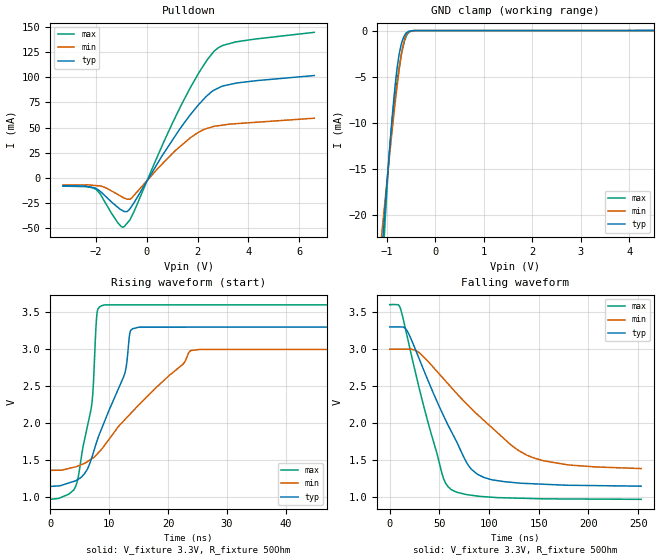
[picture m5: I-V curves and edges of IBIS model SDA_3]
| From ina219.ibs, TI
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|   3.3V SDA I/O_Open_drain Model
[Model] SDA_3   |Rload = 1k
Model_type I/O_open_drain
| Signals  SDA
Polarity   Non-Inverting
Enable   Active-Low
Vinl = 0.99
Vinh = 2.31
Vmeas = 1.65
Vref = 1.65
Cref = 0pF
Rref = 50
|   typ   min   max
|Average
C_comp   2.0039139E-10   2.3760390E-10   2.1698516E-10
|ON state
|C_comp   2.2433820e-12   2.5433970e-12   1.9431160e-12
|OFF state
|C_comp   3.9853940e-10   4.7266440e-10   4.7266440e-10
[Voltage Range]   3.3   3   3.6
[Temperature Range]   27   85   -25
[Pullup Reference]   3.3   3   3.6
[Pulldown Reference]   0   0   -0
[Power Clamp Reference]   3.3   3   3.6
[GND Clamp Reference]   0   0   0
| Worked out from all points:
|   slope of the pulldown table from 0 to 0.495 V, typ, clamps not added: 23.7 ohm
|   GND clamp passes 1 mA (typ) near -0.67 V on its own axis
|   falling waveform, V_fixture 3.3V, R_fixture 50Ohm: 20-80 % time 43.6ns typ, 72.7ns min, 30.1ns max; typ from 3.3 V to 1.15 V
|   rising waveform, V_fixture 3.3V, R_fixture 50Ohm: 20-80 % time 5.85ns typ, 11.5ns min, 2.43ns max; typ from 1.15 V to 3.3 V
[Pulldown]
|   Voltage   I(typ)   I(min)   I(max)
-3.3V     -7.794mA   -7.117mA   -8.174mA
-1.996V   -10.52mA   -7.627mA   -11.41mA
-1.14V    -29.25mA   -16.51mA   -44.63mA
-895.3mV  -33.38mA   -19.99mA   -48.61mA
-772.4mV  -33.44mA   -21.14mA   -45.1mA
-599.6mV  -28.41mA   -20.19mA   -38.58mA
630.8mV   22.96mA    14.44mA    33.51mA
1.346V    50.2mA     31.9mA     71.87mA
2.067V    73.55mA    45.72mA    105.3mA
2.644V    87.22mA    51.22mA    125.8mA
3.487V    94.06mA    53.84mA    135.1mA
6.59V     101.7mA    59.33mA    144.7mA
[GND Clamp]
|   Voltage   I(typ)   I(min)   I(max)
-3.3V     -196.9mA   -147.2mA   -279.1mA
-1.102V   -24mA      -21.89mA   -27.2mA
-1.043V   -19.69mA   -18.68mA   -21.32mA
-983.5mV  -15.54mA   -15.58mA   -16.04mA
-933.2mV  -12.15mA   -12.97mA   -12.26mA
-868.5mV  -8.1mA     -9.736mA   -8.673mA
-787.9mV  -4.013mA   -5.973mA   -5.416mA
-748.8mV  -2.626mA   -4.335mA   -4.091mA
-659.8mV  -794.9uA   -1.425mA   -1.623mA
-606.7mV  -289.9uA   -507.1uA   -723.2uA
-548.1mV  -77.69uA   -128.7uA   -218.4uA
6.59V     0A         0A         0A
[POWER Clamp]
|   SCR cell for ESD function. Effects occurr above VDD x 2
|   Voltage   I(typ)   I(min)   I(max)
-3.3V     0A         0A         0A
0V        0A         0A         0A
6.6V      0A         0A         0A
[Ramp]
R_load = 50
|   typ   min   max
dV/dt_r   1.29119/5.84889e-009  0.980788/1.14901e-008   1.57529/2.42474e-009
dV/dt_f   1.28852/4.35577e-008  0.965908/7.27422e-008   1.57486/3.01092e-008
[Falling Waveform]
V_fixture = 3.3V
V_fixture_min = 3V
V_fixture_max = 3.6V
R_fixture = 50Ohm
C_fixture = 0F
|   Time   V(typ)   V(min)   V(max)
0s        3.3V       3V         3.6V
10.79ns   3.299V     2.999V     3.548V
19.92ns   3.184V     2.999V     3.032V
29.97ns   2.859V     2.95V      2.457V
52.46ns   2.151V     2.627V     1.329V
61.66ns   1.899V     2.488V     1.108V
82.35ns   1.378V     2.196V     1.03V
102.4ns   1.24V      1.947V     1.004V
147.4ns   1.183V     1.523V     984.6mV
253.1ns   1.152V     1.39V      975.2mV
[Rising Waveform]
V_fixture = 3.3V
V_fixture_min = 3V
V_fixture_max = 3.6V
R_fixture = 50Ohm
C_fixture = 0F
|   Time   V(typ)   V(min)   V(max)
0s        1.148V     1.365V     974.5mV
4.543ns   1.235V     1.419V     1.203V
7.101ns   1.549V     1.524V     2.29V
7.971ns   1.769V     1.586V     3.5V
9.278ns   2.036V     1.708V     3.595V
12.67ns   2.674V     2.049V     3.595V
13.59ns   3.239V     2.126V     3.595V
15.07ns   3.295V     2.25V      3.595V
25.3ns    3.295V     2.994V     3.595V
253.1ns   3.3V       3V         3.6V
